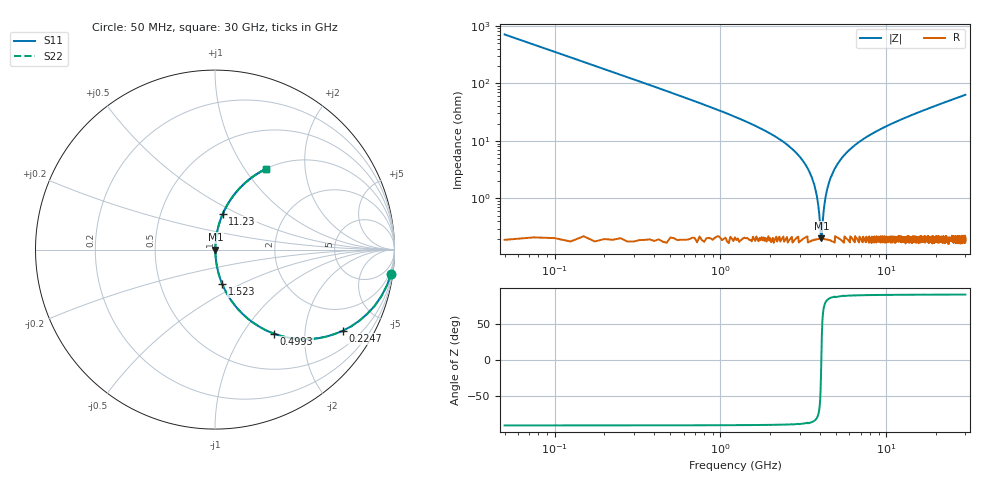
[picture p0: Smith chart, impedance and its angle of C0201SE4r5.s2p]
!	AVX Thin Film Operation 	Date: April 2014
!	Description: Accu-P® Series, Thin Film  SMD RF Capacitor
!	Part Number: 02013K4R5ABSTR
# MHZ S MA R 50
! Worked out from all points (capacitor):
!   1201 points, 50 MHz to 30 GHz, reference 50 ohm
!   read as one part in series: C = 4.5 pF near 199.8 MHz
!   lowest |Z| = 202 mohm at 4.068 GHz (marker M1)
!   series resonance near 4.059 GHz, so ESL is about 340 pH
!   S11 on the Smith chart (normalised r, x): 50 MHz: 1, -14; 224.7 MHz: 1.00, -3.14; 499.2 MHz: 1.00, -1.39; 1.523 GHz: 1.00, -0.40; 11.23 GHz: 1.00, +0.42; 30 GHz: 1.00, +1.27
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50  0.99 -8.0  0.14 81.9  0.14 81.9  0.99 -8.0
224.708  0.843 -32.5  0.537 57.4  0.537 57.4  0.843 -32.5
499.25  0.571 -55.0  0.819 34.9  0.819 34.9  0.571 -55.0
873.625  0.36 -68.6  0.931 21.1  0.931 21.1  0.36 -68.6
1522.542  0.195 -78.2  0.979 11.3  0.979 11.3  0.195 -78.2
2670.625  0.075 -84.2  0.995 4.3  0.995 4.3  0.075 -84.2
3294.583  0.037 -84.9  0.997 2.1  0.997 2.1  0.037 -84.9
3668.958  0.018 -82.7  0.998 1.0  0.998 1.0  0.018 -82.7
3793.75  0.012 -79.9  0.998 0.7  0.998 0.7  0.012 -79.9
3968.458  0.00437 -63.3  0.998 0.2  0.998 0.2  0.00437 -63.3
4068.292  0.001989 11.8  0.998 -0.0  0.998 -0.0  0.001989 11.8
4168.125  0.005019 66.9  0.998 -0.3  0.998 -0.3  0.005019 66.9
4317.875  0.011 79.1  0.998 -0.6  0.998 -0.6  0.011 79.1
4492.583  0.018 82.7  0.998 -1.0  0.998 -1.0  0.018 82.7
5041.667  0.038 84.9  0.997 -2.2  0.997 -2.2  0.038 84.9
6838.667  0.095 83.4  0.994 -5.4  0.994 -5.4  0.095 83.4
10058.29  0.178 79.2  0.982 -10.2  0.982 -10.2  0.178 79.2
11231.33  0.205 77.6  0.977 -11.8  0.977 -11.8  0.205 77.6
15025  0.286 73.0  0.956 -16.6  0.956 -16.6  0.286 73.0
20016.67  0.38 67.4  0.923 -22.4  0.923 -22.4  0.38 67.4
25033.29  0.463 62.2  0.885 -27.6  0.885 -27.6  0.463 62.2
30000  0.534 57.6  0.844 -32.3  0.844 -32.3  0.534 57.6
